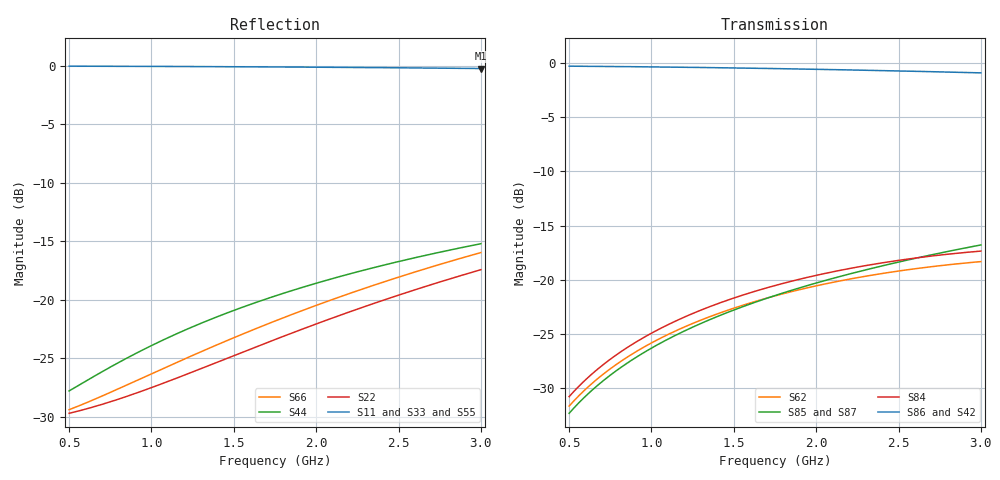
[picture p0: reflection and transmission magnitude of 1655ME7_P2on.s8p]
! Created Fri Dec 10 20:28:06 2010
# hz S db R 50
! 8 Port Network Data from SP1.SP block
! freq  dbS11  angS11  dbS12  angS12  dbS13  angS13  dbS14  angS14
!  dbS15  angS15  dbS16  angS16  dbS17  angS17  dbS18  angS18
!  dbS21  angS21  dbS22  angS22  dbS23  angS23  dbS24  angS24
!  dbS25  angS25  dbS26  angS26  dbS27  angS27  dbS28  angS28
!  dbS31  angS31  dbS32  angS32  dbS33  angS33  dbS34  angS34
!  dbS35  angS35  dbS36  angS36  dbS37  angS37  dbS38  angS38
!  dbS41  angS41  dbS42  angS42  dbS43  angS43  dbS44  angS44
!  dbS45  angS45  dbS46  angS46  dbS47  angS47  dbS48  angS48
!  dbS51  angS51  dbS52  angS52  dbS53  angS53  dbS54  angS54
!  dbS55  angS55  dbS56  angS56  dbS57  angS57  dbS58  angS58
!  dbS61  angS61  dbS62  angS62  dbS63  angS63  dbS64  angS64
!  dbS65  angS65  dbS66  angS66  dbS67  angS67  dbS68  angS68
!  dbS71  angS71  dbS72  angS72  dbS73  angS73  dbS74  angS74
!  dbS75  angS75  dbS76  angS76  dbS77  angS77  dbS78  angS78
!  dbS81  angS81  dbS82  angS82  dbS83  angS83  dbS84  angS84
!  dbS85  angS85  dbS86  angS86  dbS87  angS87  dbS88  angS88
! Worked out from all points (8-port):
!   251 points, 500 MHz to 3 GHz, reference 50 ohm
!   strongest paths, dB at 500 MHz, 1.12 GHz, 1.75 GHz, 2.38 GHz, 3 GHz:
!     S86: -0.3, -0.4, -0.5, -0.7, -0.9
!     S42: -0.3, -0.4, -0.5, -0.7, -0.9
!     S84: -30.8, -24.0, -20.5, -18.5, -17.4
!     S85: -32.3, -25.3, -21.4, -18.8, -16.8
!     S62: -31.6, -24.9, -21.5, -19.5, -18.3
!     S87: -32.4, -25.4, -21.5, -18.8, -16.7
!   lowest |S11| = -0.2 dB at 3 GHz (marker M1), VSWR 75.60, Z = 21.8 - j282 ohm
!   |S11| at or under -10 dB: nowhere
